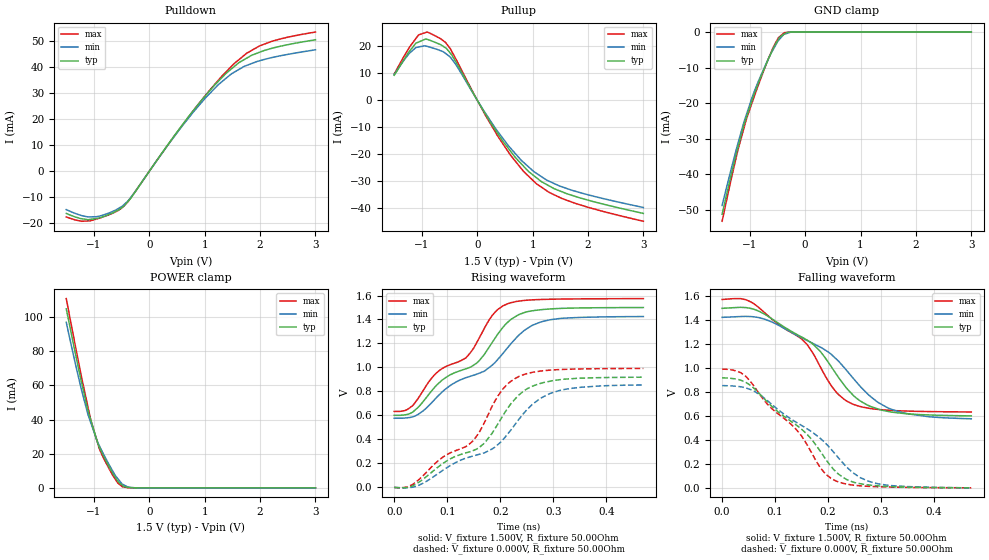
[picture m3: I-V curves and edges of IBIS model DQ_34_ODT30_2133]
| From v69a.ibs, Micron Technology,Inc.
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| MODEL DQ_34_ODT30_2133 (34 Ohm Data I/O with 30ohm ODT, 1866/2133 Mbps)
[Model]   DQ_34_ODT30_2133
Model_type   I/O
Vinl = 625.000mV
Vinh = 875.000mV
Vmeas = 750.000mV
Vref = 750.000mV
Cref = 0.0pF
Rref = 25.000Ohm
|   typ   min   max
C_comp   1.19pF   1.04pF   1.35pF
| Note: C_comp changes when the ODT circuit is enabled.
[Model Spec]
| Input threshold voltage corners
Vinl   0.6250V   0.5875V   0.6625V
Vinh   0.8750V   0.8375V   0.9125V
| Measurement voltage corners
Vmeas   0.7500V   0.7125V   0.7875V
| Timing spec test load voltage corners
Vref   0.7500V   0.7125V   0.7875V
[Receiver Thresholds]
Vth   =  0.750V
Vth_min  =  0.735V
Vth_max  =  0.765V
Vinh_ac  =  0.125V
Vinh_dc  =  0.100V
Vinl_ac  = -0.125V
Vinl_dc  = -0.100V
Tslew_ac =  5.000ns |Not specified, so set to high value
Threshold_sensitivity = 0.50
Reference_supply Pullup_ref
[Voltage Range]   1.5000V   1.4250V   1.5750V
[Pullup Reference]   1.5000V   1.4250V   1.5750V
| Junction Temperature (Ambient temp is 35C typ, 95C min, 0C max)
[Temperature Range]   50.0   110.0   0.0
[Add Submodel]
| Submodel Name   Mode
30ohm_ODT_2133   Non-Driving
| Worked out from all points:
|   slope of the pulldown table from 0 to 0.225 V, typ, clamps not added: 32.5 ohm
|   slope of the pullup table from 0 to 0.225 V, typ, clamps not added: 28.9 ohm
|   GND clamp passes 1 mA (typ) near -0.42 V on its own axis
|   POWER clamp passes 1 mA (typ) near -0.47 V on its own axis
|   falling waveform, V_fixture 1.500V, R_fixture 50.00Ohm: 20-80 % time 120ps typ, 135ps min, 111ps max; typ from 1.5 V to 0.601 V
|   rising waveform, V_fixture 1.500V, R_fixture 50.00Ohm: 20-80 % time 136ps typ, 153ps min, 121ps max; typ from 0.601 V to 1.5 V
|   rising waveform, V_fixture 0.000V, R_fixture 50.00Ohm: 20-80 % time 141ps typ, 157ps min, 124ps max; typ from 0 V to 0.919 V
|   falling waveform, V_fixture 0.000V, R_fixture 50.00Ohm: 20-80 % time 123ps typ, 138ps min, 112ps max; typ from 0.919 V to 0 V
[Pulldown]
|   Voltage   I(typ)   I(min)   I(max)
-1.5V     -16.29mA   -14.8mA    -17.64mA
-1.105V   -18.68mA   -17.63mA   -19.15mA
-880mV    -17.85mA   -17.19mA   -17.94mA
-555mV    -14.94mA   -14.32mA   -15.02mA
-385mV    -11.64mA   -11.48mA   -11.69mA
795mV     23.36mA    22.81mA    23.33mA
1.02V     29.25mA    28.38mA    29.37mA
1.39V     37.78mA    35.88mA    38.36mA
1.755V    43.51mA    40.72mA    45.39mA
1.99V     45.82mA    42.53mA    48.26mA
2.365V    48.13mA    44.46mA    50.94mA
3V        50.62mA    46.76mA    53.61mA
[GND Clamp]
|   Voltage   I(typ)   I(min)   I(max)
-1.5V     -51.33mA   -48.85mA   -53.31mA
-1.225V   -33.17mA   -31.96mA   -33.91mA
-1.11V    -26.38mA   -25.59mA   -27.31mA
-1.06V    -24mA      -23.21mA   -24.46mA
-955mV    -19.04mA   -18.24mA   -19.74mA
-855mV    -14.8mA    -14.26mA   -15.35mA
-575mV    -4.569mA   -4.842mA   -4.255mA
-455mV    -1.373mA   -1.876mA   -1.232mA
-380mV    -600.5uA   -637.3uA   -211uA
-330mV    -105.7uA   -382.3uA   -79.03uA
-165mV    -2.061uA   -3.044uA   0A
3V        0A         0A         0A
[Pullup]
|   Voltage   I(typ)   I(min)   I(max)
-1.5V     9.275mA    9.623mA    9.786mA
-1.225V   18.22mA    17.48mA    19.7mA
-1.06V    21.64mA    19.81mA    24.28mA
-905mV    22.64mA    20.04mA    25.36mA
-660mV    20.66mA    18.41mA    22.85mA
-490mV    17.59mA    16.11mA    19.25mA
-390mV    14.39mA    13.4mA     15.49mA
375mV     -12.49mA   -11.73mA   -13.49mA
700mV     -21.55mA   -20.1mA    -22.95mA
1.065V    -28.73mA   -27.11mA   -30.95mA
1.755V    -35.63mA   -33.71mA   -38.2mA
3V        -42.05mA   -39.85mA   -44.97mA
[POWER Clamp]
|   Voltage   I(typ)   I(min)   I(max)
-1.5V     104.9mA    96.95mA    110.8mA
-1.305V   73.96mA    68.35mA    78.05mA
-1.11V    45.47mA    43.15mA    47.59mA
-1.06V    40.01mA    38.39mA    40.06mA
-955mV    28.63mA    28.51mA    28.54mA
-905mV    24.01mA    24.84mA    23.06mA
-660mV    8.35mA     9.771mA    7.255mA
-570mV    3.953mA    5.39mA     2.853mA
-490mV    1.557mA    2.191mA    712uA
-385mV    314.2uA    439.4uA    73.92uA
-265mV    10.67uA    38.19uA    0A
3V        0A         0A         0A
[Ramp]
R_load = 50.00Ohm
|   typ   min   max
dV/dt_r   551.471mV/140.807ps 512.490mV/156.929ps 595.210mV/123.769ps
dV/dt_f   539.233mV/119.683ps 508.442mV/135.202ps 564.059mV/110.832ps
[Falling Waveform]
V_fixture = 1.500V
V_fixture_min = 1.425V
V_fixture_max = 1.575V
R_fixture = 50.00Ohm
|   Time   V(typ)   V(min)   V(max)
0s        1.5V       1.425V     1.574V
55ps      1.498V     1.431V     1.551V
95ps      1.409V     1.383V     1.406V
165ps     1.221V     1.221V     1.168V
185ps     1.141V     1.177V     1.013V
210ps     985.3mV    1.098V     828.9mV
245ps     783.8mV    927.2mV    702.2mV
280ps     680mV      762.7mV    662.4mV
320ps     632.7mV    655.1mV    646.8mV
470ps     601.2mV    577.1mV    634mV
[Rising Waveform]
V_fixture = 1.500V
V_fixture_min = 1.425V
V_fixture_max = 1.575V
R_fixture = 50.00Ohm
|   Time   V(typ)   V(min)   V(max)
0s        601.2mV    577.1mV    634mV
45ps      667.2mV    608.1mV    740.8mV
80ps      853mV      750.3mV    955.6mV
135ps     988.6mV    914.4mV    1.079V
160ps     1.055V     951.7mV    1.242V
185ps     1.21V      1.02V      1.435V
210ps     1.36V      1.144V     1.524V
245ps     1.457V     1.308V     1.559V
280ps     1.483V     1.384V     1.567V
470ps     1.5V       1.425V     1.574V
[Rising Waveform]
V_fixture = 0.000V
V_fixture_min = 0.000V
V_fixture_max = 0.000V
R_fixture = 50.00Ohm
|   Time   V(typ)   V(min)   V(max)
0s        -16.13uV   137.9uV    159.9uV
35ps      13.83mV    2.175mV    25.31mV
90ps      194.5mV    137.6mV    247mV
145ps     300mV      257.3mV    373.5mV
170ps     368.6mV    288mV      539.7mV
205ps     598.5mV    396.6mV    820.8mV
235ps     770.8mV    566.8mV    924.6mV
275ps     866.4mV    739.9mV    969.5mV
315ps     899.5mV    811.9mV    983.2mV
470ps     919.1mV    854.3mV    992.2mV
[Falling Waveform]
V_fixture = 0.000V
V_fixture_min = 0.000V
V_fixture_max = 0.000V
R_fixture = 50.00Ohm
|   Time   V(typ)   V(min)   V(max)
0s        919.1mV    854.3mV    992.2mV
45ps      880.3mV    834.5mV    930.3mV
85ps      719.5mV    730.1mV    701.6mV
135ps     540.6mV    560.7mV    511mV
160ps     448.2mV    493.8mV    363mV
185ps     307.2mV    414.3mV    170mV
215ps     133.2mV    273.5mV    57.05mV
250ps     43.92mV    116.3mV    21.15mV
290ps     18.26mV    38.31mV    9.758mV
470ps     -16.13uV   137.9uV    159.9uV
